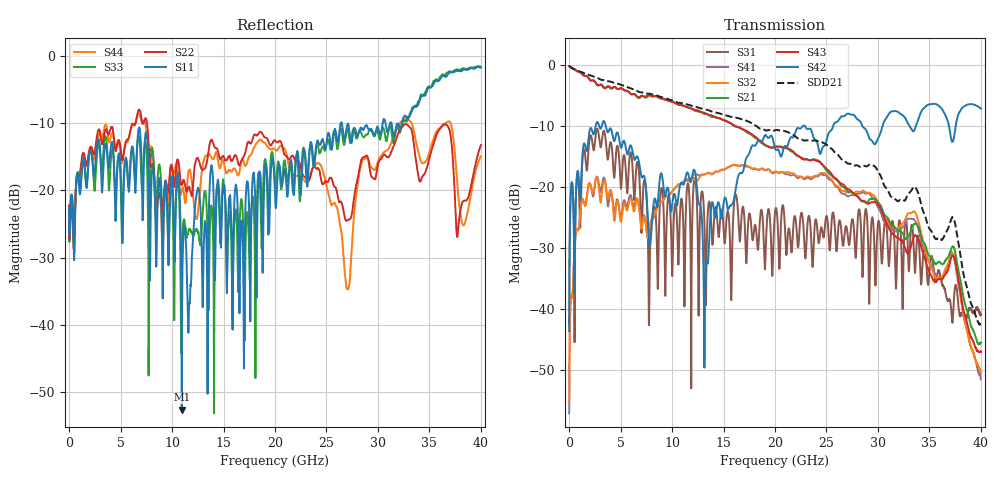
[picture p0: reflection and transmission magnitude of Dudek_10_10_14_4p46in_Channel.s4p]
! Created Thu Oct 09 16:29:54 2014
# hz S ma R 50
! 4 Port Network Data from SP1.SP block
! freq  magS11  angS11  magS12  angS12  magS13  angS13  magS14  angS14
!  magS21  angS21  magS22  angS22  magS23  angS23  magS24  angS24
!  magS31  angS31  magS32  angS32  magS33  angS33  magS34  angS34
!  magS41  angS41  magS42  angS42  magS43  angS43  magS44  angS44
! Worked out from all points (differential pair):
!   4001 points, 10 kHz to 40 GHz, reference 50 ohm
!   strongest paths, dB at 10 kHz, 10 GHz, 20 GHz, 30 GHz, 40 GHz:
!     S42: -43.7, -23.0, -13.6, -12.0, -7.1
!     S43: -0.1, -6.0, -13.3, -22.9, -47.0
!     S21: -0.1, -6.0, -13.4, -22.5, -45.6
!     S32: -55.5, -20.7, -17.5, -22.5, -50.5
!     S41: -57.2, -20.8, -17.6, -23.4, -51.6
!     S31: -42.5, -34.3, -24.2, -26.0, -41.0
!   taken as a pair (ports 3,1 in; 4,2 out), SDD21 dB: -0.1, -5.8, -10.7, -17.4, -42.8
!   lowest |S11| = -52.6 dB at 10.94 GHz (marker M1), VSWR 1.00, Z = 50.2 + j0.0112 ohm
!   |S11| at or under -10 dB: start of sweep to 26.4 GHz; 26.49 GHz to 30.47 GHz (3.987 GHz wide, 14 % of centre); 31.31 GHz to 32.34 GHz (1.025 GHz wide, 3.22 % of centre)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
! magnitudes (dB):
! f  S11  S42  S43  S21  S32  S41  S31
! 10 kHz  -22.7  -43.7  -0.1  -0.1  -55.5  -57.2  -42.5
! 1.94 GHz  -14.8  -11.2  -2.2  -2.2  -19.4  -19.4  -12.7
! 10.94 GHz  -52.6  -19.3  -6.6  -6.5  -19.4  -19.4  -22.0
! 13.25 GHz  -24.8  -34.4  -8.0  -7.9  -17.9  -17.9  -36.2
! 27.07 GHz  -10.1  -7.9  -20.3  -20.7  -20.9  -21.5  -28.0
! 33.53 GHz  -7.5  -10.7  -28.1  -26.1  -24.0  -25.4  -32.1
! 40 GHz  -1.8  -7.1  -47.0  -45.6  -50.5  -51.6  -41.0
